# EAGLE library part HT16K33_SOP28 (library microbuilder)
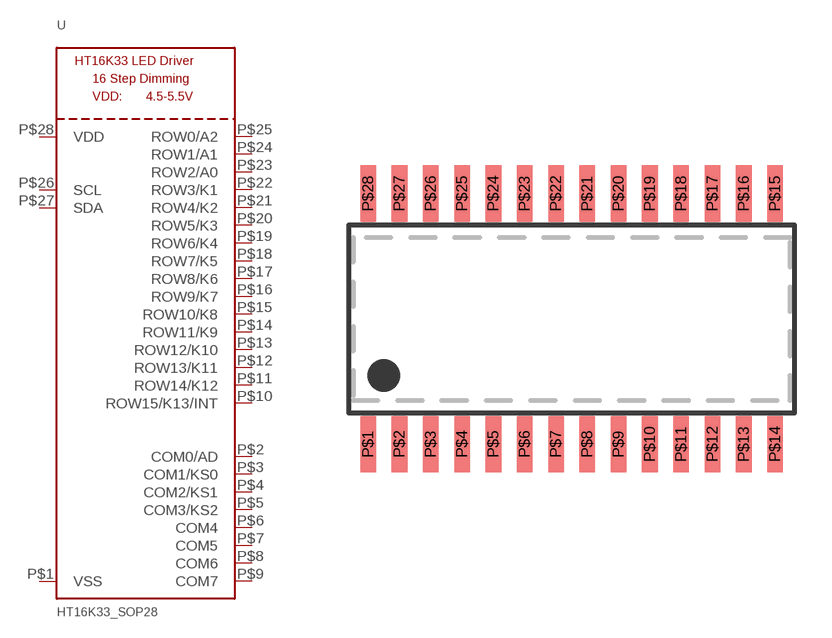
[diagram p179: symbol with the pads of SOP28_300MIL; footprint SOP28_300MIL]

Designator prefix U

## HT16K33_SOP28  [SOP28_300MIL]
P$1  VSS
P$2  COM0/AD
P$3  COM1/KS0
P$4  COM2/KS1
P$5  COM3/KS2
P$6  COM4
P$7  COM5
P$8  COM6
P$9  COM7
P$10  ROW15/K13/INT
P$11  ROW14/K12
P$12  ROW13/K11
P$13  ROW12/K10
P$14  ROW11/K9
P$15  ROW10/K8
P$16  ROW9/K7
P$17  ROW8/K6
P$18  ROW7/K5
P$19  ROW6/K4
P$20  ROW5/K3
P$21  ROW4/K2
P$22  ROW3/K1
P$23  ROW2/A0
P$24  ROW1/A1
P$25  ROW0/A2
P$26  SCL
P$27  SDA
P$28  VDD

## Footprint SOP28_300MIL (pad centres in mm)
smd 0.635 x 2.286: P$1 -8.255,-5.08; P$2 -6.985,-5.08; P$3 -5.715,-5.08; P$4 -4.445,-5.08; P$5 -3.175,-5.08; P$6 -1.905,-5.08; P$7 -0.635,-5.08; P$8 0.635,-5.08; P$9 1.905,-5.08; P$10 3.175,-5.08; P$11 4.445,-5.08; P$12 5.715,-5.08; P$13 6.985,-5.08; P$14 8.255,-5.08; P$15 8.255,5.08; P$16 6.985,5.08; P$17 5.715,5.08; P$18 4.445,5.08; P$19 3.175,5.08; P$20 1.905,5.08; P$21 0.635,5.08; P$22 -0.635,5.08; P$23 -1.905,5.08; P$24 -3.175,5.08; P$25 -4.445,5.08; P$26 -5.715,5.08; P$27 -6.985,5.08; P$28 -8.255,5.08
